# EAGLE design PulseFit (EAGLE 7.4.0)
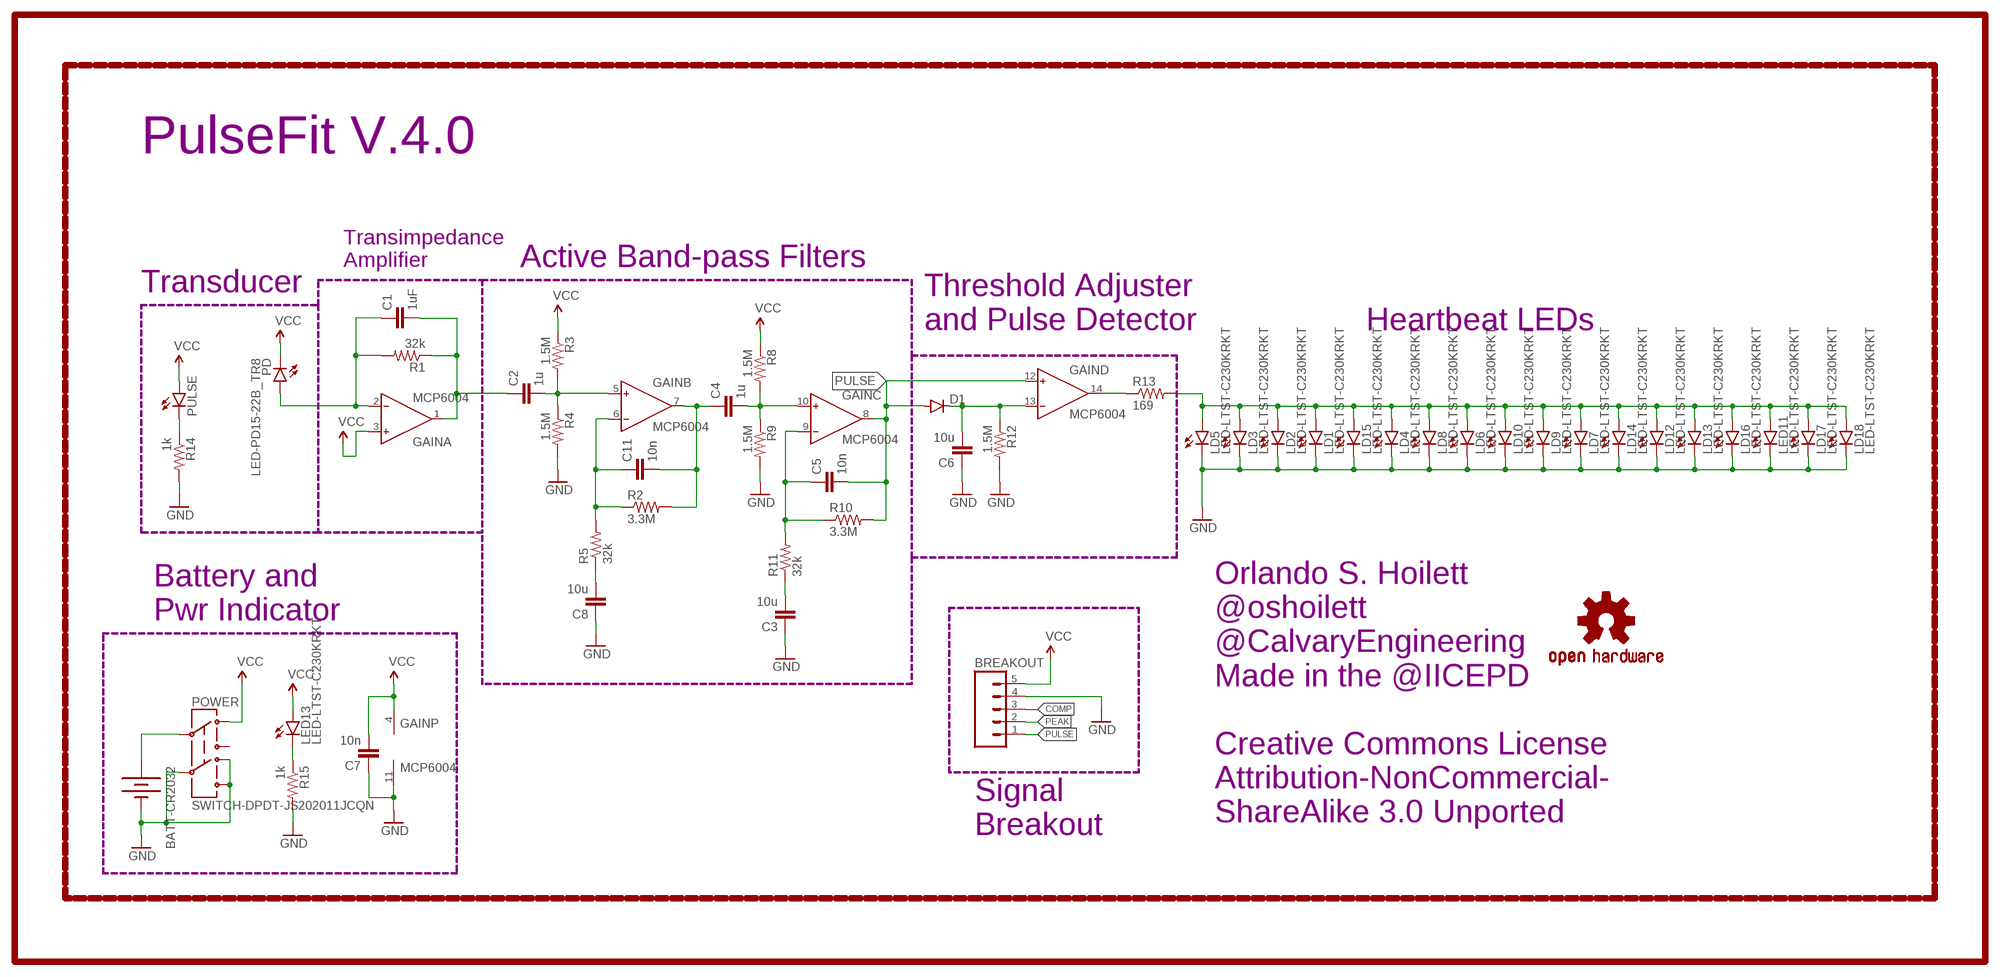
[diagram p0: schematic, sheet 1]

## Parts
BATT-CR2032  BATTERY20SMD  [BATTCON_20MM]
BREAKOUT  M05NO_SILK  [1X05_NO_SILK]
C1  1uF  C-EUC0402  [C0402]
C2  1u  C-EUC0402  [C0402]
C3  10u  C-EUC0805  [C0805]
C4  1u  C-EUC0402  [C0402]
C5  10n  C-EUC0402  [C0402]
C6  10u  C-EUC0805  [C0805]
C7  10n  C-EUC0402  [C0402]
C8  10u  C-EUC0805  [C0805]
C11  10n  C-EUC0402  [C0402]
D1  250mA/100V  DIODEBAS16  [SOD-323]
GAIN  MCP6004  AD8609RU  [TSSOP14]
LD1  LED-LTST-C230KRKT  [LED-1206-BOTTOM]
LD2  LED-LTST-C230KRKT  [LED-1206-BOTTOM]
LD3  LED-LTST-C230KRKT  [LED-1206-BOTTOM]
LD4  LED-LTST-C230KRKT  [LED-1206-BOTTOM]
LD5  LED-LTST-C230KRKT  [LED-1206-BOTTOM]
LD6  LED-LTST-C230KRKT  [LED-1206-BOTTOM]
LD7  LED-LTST-C230KRKT  [LED-1206-BOTTOM]
LD8  LED-LTST-C230KRKT  [LED-1206-BOTTOM]
LD9  LED-LTST-C230KRKT  [LED-1206-BOTTOM]
LD10  LED-LTST-C230KRKT  [LED-1206-BOTTOM]
LD12  LED-LTST-C230KRKT  [LED-1206-BOTTOM]
LD13  LED-LTST-C230KRKT  [LED-1206-BOTTOM]
LD14  LED-LTST-C230KRKT  [LED-1206-BOTTOM]
LD15  LED-LTST-C230KRKT  [LED-1206-BOTTOM]
LD16  LED-LTST-C230KRKT  [LED-1206-BOTTOM]
LD17  LED-LTST-C230KRKT  [LED-1206-BOTTOM]
LD18  LED-LTST-C230KRKT  [LED-1206-BOTTOM]
LED11  LED-LTST-C230KRKT  [LED-1206-BOTTOM]
LED13  LED-LTST-C230KRKT  [LED-1206-BOTTOM]
LOGO1  OSHW-LOGOS  [OSHW-LOGO-S]
PD  LED-PD15-22B_TR8  [LED-PD15-22B_TR8]
POWER  SWITCH-DPDT-JS202011JCQN  [J-LEAD]
PULSE  LED0603  [LED-0603]
R1  32k  R-US_R0402  [R0402]
R2  3.3M  R-US_R0402  [R0402]
R3  1.5M  R-US_R0402  [R0402]
R4  1.5M  R-US_R0402  [R0402]
R5  32k  R-US_R0402  [R0402]
R8  1.5M  R-US_R0402  [R0402]
R9  1.5M  R-US_R0402  [R0402]
R10  3.3M  R-US_R0402  [R0402]
R11  32k  R-US_R0402  [R0402]
R12  1.5M  R-US_R0402  [R0402]
R13  169  R-US_R0402  [R0402]
R14  1k  R-US_R0402  [R0402]
R15  1k  R-US_R0402  [R0402]

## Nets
ANODE: LD1.A LD2.A LD3.A LD4.A LD5.A LD6.A LD7.A LD8.A LD9.A LD10.A LD12.A LD13.A LD14.A LD15.A LD16.A LD17.A LD18.A LED11.A R13.2
COMP: BREAKOUT.3 GAIN.14(D:OUT) R13.1
GND: BATT-CR2032.2(-) BREAKOUT.4 C3.1 C6.1 C7.1 C8.1 GAIN.11(P:V-) LD1.C LD2.C LD3.C LD4.C LD5.C LD6.C LD7.C LD8.C LD9.C LD10.C LD12.C LD13.C LD14.C LD15.C LD16.C LD17.C LD18.C LED11.C POWER.4 POWER.5 POWER.6 R4.2 R9.2 R12.2 R14.2 R15.2
N$1: C1.1 GAIN.2(A:IN-) PD.A-1(A) PD.A-2(A) R1.2
N$2: C1.2 C2.1 GAIN.1(A:OUT) R1.1
N$3: C4.2 GAIN.10(C:IN+) R8.2 R9.1
N$4: C2.2 GAIN.5(B:IN+) R3.2 R4.1
N$5: BATT-CR2032.1(+) POWER.2
N$6: C3.2 R11.1
N$8: C5.1 GAIN.9(C:IN-) R10.1 R11.2
N$9: PULSE.C R14.1
N$10: C11.1 GAIN.6(B:IN-) R2.1 R5.2
N$11: C4.1 C11.2 GAIN.7(B:OUT) R2.2
N$12: LED13.C R15.1
N$14: C8.2 R5.1
PEAK: BREAKOUT.2 C6.2 D1.C GAIN.13(D:IN-) R12.1
PULSE: BREAKOUT.1 C5.2 D1.A GAIN.8(C:OUT) GAIN.12(D:IN+) R10.2
VCC: BREAKOUT.5 C7.2 GAIN.3(A:IN+) GAIN.4(P:V+) LED13.A PD.C-1(C) PD.C-2(C) POWER.1 PULSE.A R3.1 R8.1
Unconnected: POWER.3

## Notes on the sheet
- PulseFit V.4.0
- Transimpedance
  Amplifier
- Active Band-pass Filters
- Transducer
- Threshold Adjuster
  and Pulse Detector
- Heartbeat LEDs
- Battery and
  Pwr Indicator
- Orlando S. Hoilett
  @oshoilett
  @CalvaryEngineering
  Made in the @IICEPD
  
  Creative Commons License
  Attribution-NonCommercial-
  ShareAlike 3.0 Unported
- Signal
  Breakout

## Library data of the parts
BATT-CR2032 = SparkFun-Electromechanical:BATTERY: Battery Holders
BREAKOUT = SparkFun-Connectors:M05: Header 5 Standard 5-pin 0.1" header. Use with straight break away headers (SKU : PRT-00116), right angle break away headers (PRT-00553), swiss pins (PRT-00743), machine pins (PRT-00117), and female headers (PRT-00115). Molex polarized connector foot print use with SKU : PRT-08230 with associated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
C1-C8 C11 = resistor:C-EU: CAPACITOR, European symbol
D1 = SparkFun-DiscreteSemi:DIODE: Diode; PROD_ID: DIO-09646
GAIN = analog-devices:AD8609: Precision Micropower, Low Noise CMOS, Rail-to-Rail Input/Output Operational Amplifiers Source: http://www.analog.com/static/imported-files/data_sheets/AD8603_8607_8609.pdf; MF: ALTERA CORPORATION; MPN: AD8609ARUZ; OC_FARNELL: 1464994; OC_NEWARK: 59K6934
LD1-LD10 LD12-LD18 LED11 LED13 = Orlando:LED-LTST-C230KRKT
LOGO1 = SparkFun-Aesthetics:OSHW-LOGO: Open Source Hardware Logo This logo indicates the piece of hardware it is found on incorporates a OSHW license and/or adheres to the definition of open source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
PD = Orlando:LED-PD15-22B_TR8
POWER = SparkFun-Electromechanical:SWITCH-DPDT-JS202011JCQN
PULSE = SparkFun-LED:LED: LEDs
R1-R5 R8-R15 = resistor:R-US_: RESISTOR, American symbol

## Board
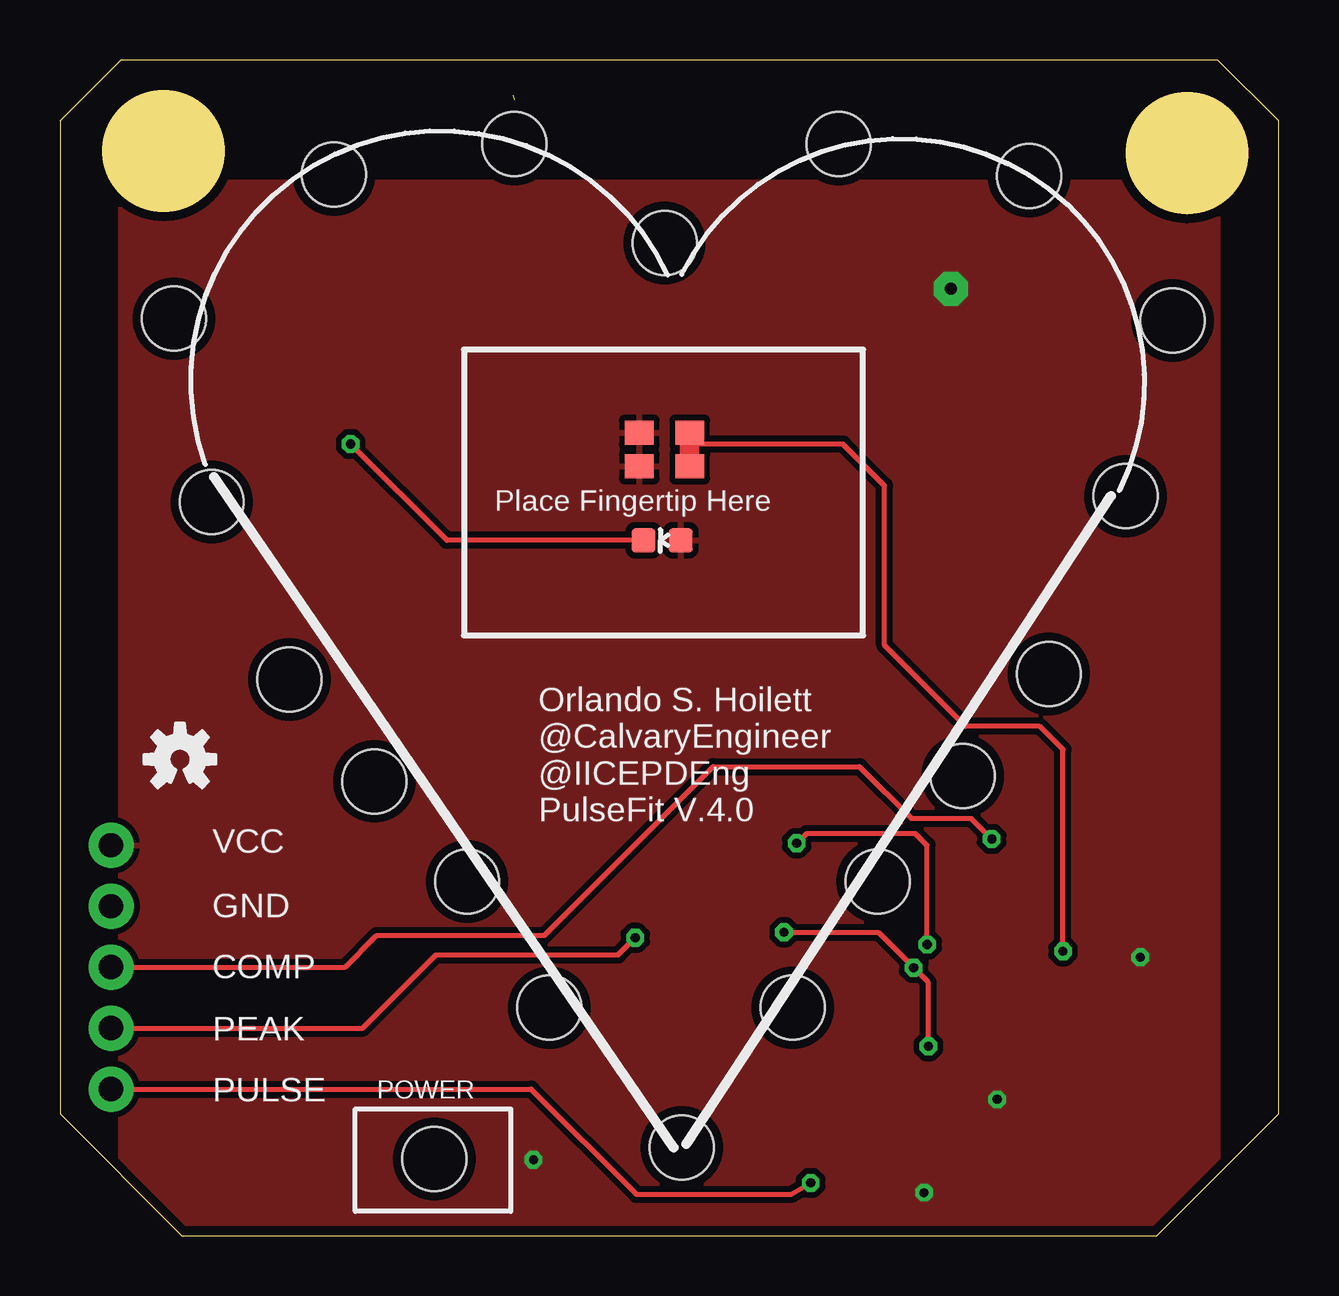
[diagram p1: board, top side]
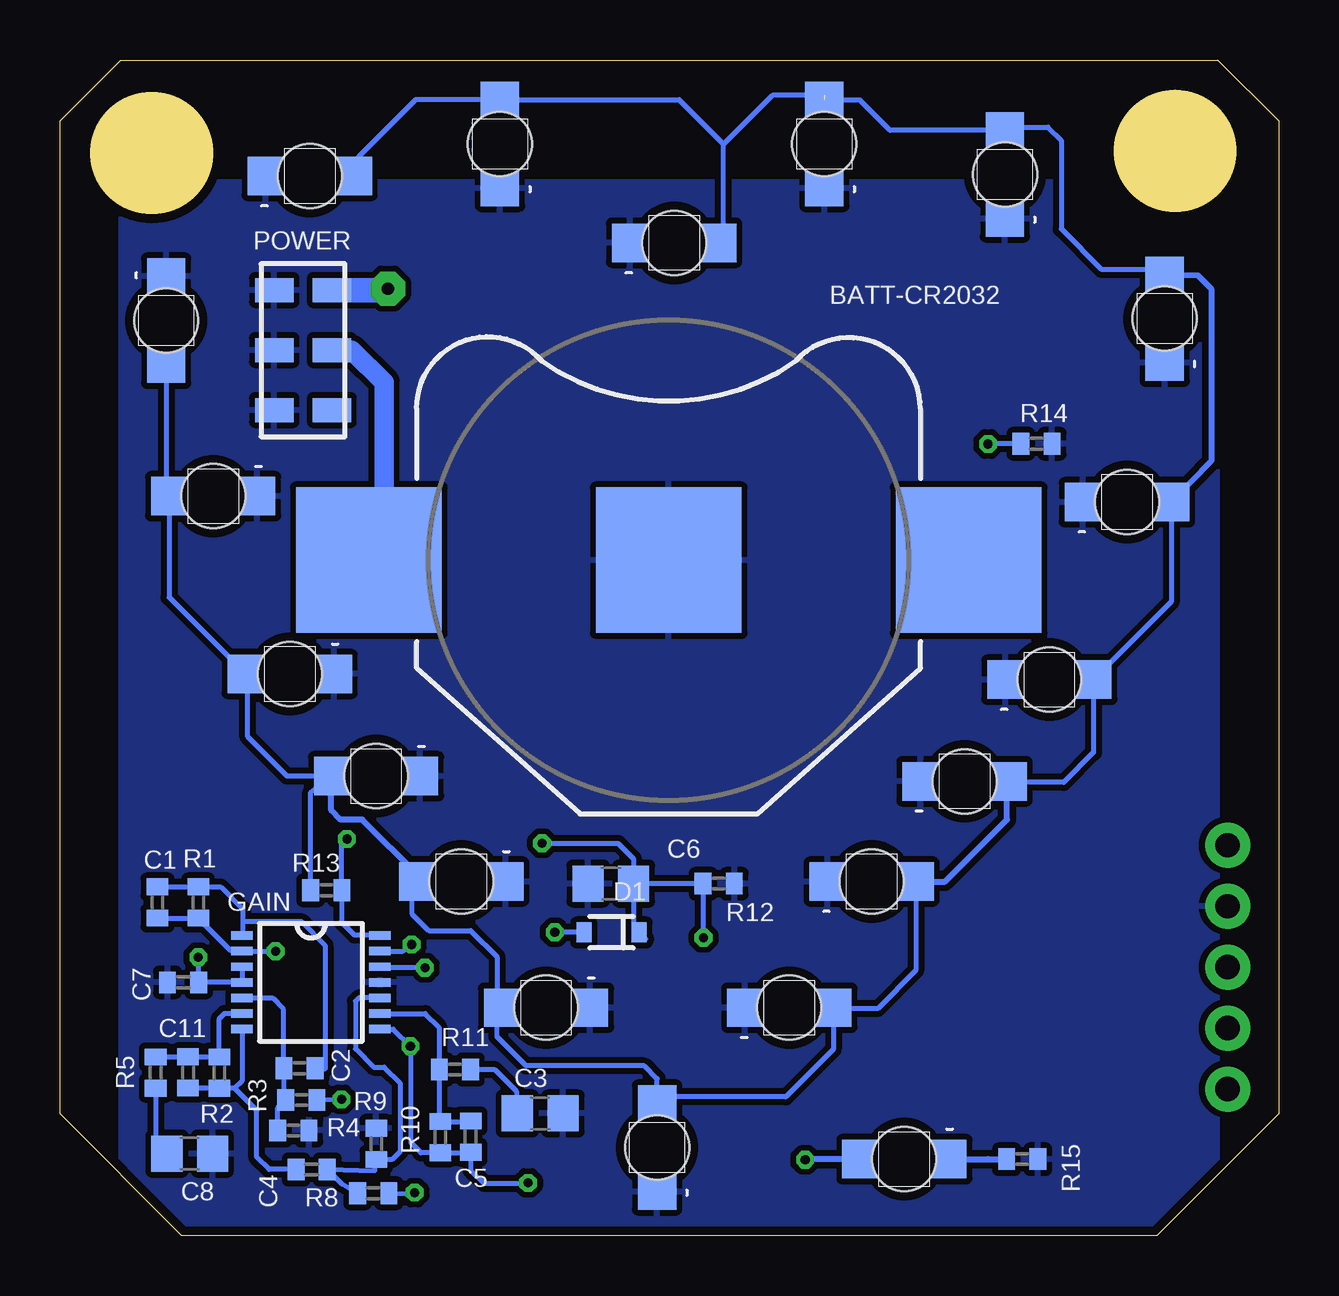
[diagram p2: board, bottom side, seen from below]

Size 50.8 x 49 mm. Coordinates in mm from the lower left corner, seen from the top.
Outline: 4.29,45.21 4.34,45.21
Outline: 46.95,45.12 47,45.12
Outline: 5.08,0 45.72,0 50.8,5.08 50.8,46.46 48.26,49 2.54,49 0,46.46 0,5.08 5.08,0
Copper layers (1*16): Top 0.0356mm / dielectric 1.5011mm / Bottom 0.0356mm
Design rules "LaenPCBOrder": minimum track width 6mil, minimum drill 13mil, track to track 6mil, track to pad 6mil, pad to pad 6mil, via to via 6mil, smd to smd 6mil, copper to edge 15mil, drill to drill 6mil, minimum pad ring 7mil, minimum via ring 7mil, stop-mask expansion 3mil, vias tented up to drill 0mil, thermal gap 10mil

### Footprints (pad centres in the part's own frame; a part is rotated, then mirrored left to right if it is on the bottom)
BATTCON_20MM = smd 6.07 x 6.07: 1 -12.5,0; 2 0,0; 3 12.5,0
1X05_NO_SILK = drill 1.016 pad 1.88: 1 0,0; 2 2.54,0; 3 5.08,0; 4 7.62,0; 5 10.16,0
C0402 = smd 0.7 x 0.9: 1 -0.65,0; 2 0.65,0
C0805 = smd 1.3 x 1.5: 1 -0.95,0; 2 0.95,0
SOD-323 = smd 0.63 x 0.83: A 1.15,0; C -1.15,0
TSSOP14 = smd 0.9 x 0.35: 1 -2.875,1.95; 2 -2.875,1.3; 3 -2.875,0.65; 4 -2.875,0; 5 -2.875,-0.65; 6 -2.875,-1.3; 7 -2.875,-1.95; 8 2.875,-1.95; 9 2.875,-1.3; 10 2.875,-0.65; 11 2.875,0; 12 2.875,0.65; 13 2.875,1.3; 14 2.875,1.95
LED-1206-BOTTOM = smd 1.5 x 1.6: A -1.841,0; C 1.841,0 | hole 2.667: 0,0
LED-PD15-22B_TR8 = smd 1.2 x 1: A-1 -1.05,0.7; A-2 -1.05,-0.7; C-1 1.05,0.7; C-2 1.05,-0.7
J-LEAD = smd 1 x 1.6: 1 -2.5,1.2; 2 0,1.2; 3 2.5,1.2; 4 -2.5,-1.2; 5 0,-1.2; 6 2.5,-1.2
LED-0603 = smd 1 x 1: A 0,-0.677; C 0,0.877
R0402 = smd 0.7 x 0.9: 1 -0.65,0; 2 0.65,0

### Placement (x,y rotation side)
BATT-CR2032  25.43,28.16 0 bottom
BREAKOUT  2.13,6.12 90 top
C1  46.74,13.89 90 bottom
C2  40.82,6.99 180 bottom
C3  30.78,5.11 180 bottom
C4  40.31,2.77 0 bottom
C5  33.68,4.14 270 bottom
C6  27.84,14.68 0 bottom
C7  45.67,10.57 0 bottom
C8  45.39,3.43 180 bottom
C11  45.46,6.81 270 bottom
D1  27.81,12.65 180 bottom
GAIN  40.34,10.57 0 bottom
LD1  25.2,41.38 180 bottom
LD2  32.46,45.5 270 bottom
LD3  40.39,44.16 180 bottom
LD4  46.37,38.14 90 bottom
LD5  44.41,30.82 0 bottom
LD6  41.22,23.41 0 bottom
LD7  37.62,19.16 0 bottom
LD8  34.08,14.77 0 bottom
LD9  30.54,9.51 0 bottom
LD10  25.91,3.68 270 bottom
LD12  16.97,14.77 180 bottom
LD13  13.1,18.94 180 bottom
LD14  9.56,23.18 180 bottom
LD15  6.32,30.58 180 bottom
LD16  4.75,38.22 270 bottom
LD17  11.41,44.23 270 bottom
LD18  18.94,45.5 270 bottom
LED11  20.4,9.51 180 bottom
LED13  15.61,3.2 0 bottom
LOGO1  5,19.86 0 top
PD  25.2,32.77 180 top
POWER  40.67,36.91 270 bottom
PULSE  25.2,28.98 90 top
R1  45.03,13.89 270 bottom
R2  44.16,6.8 270 bottom
R3  40.74,5.66 180 bottom
R4  41.07,4.39 0 bottom
R5  46.81,6.81 90 bottom
R8  37.74,1.78 180 bottom
R9  37.62,3.84 90 bottom
R10  34.95,4.11 270 bottom
R11  34.34,6.93 180 bottom
R12  23.34,14.68 0 bottom
R13  39.7,14.4 180 bottom
R14  10.1,33.01 0 bottom
R15  10.69,3.2 0 bottom

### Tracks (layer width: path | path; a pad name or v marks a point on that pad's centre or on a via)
ANODE  (1 unrouted)
  Bottom 0.203: R13.2 40.35,18.48 LD7.A 41.33,19.16 42.98,20.8 42.98,22.71 43.02,22.75 | 23.11,41.38 LD1.A 23.14,41.39 23.14,45.49 | LD13.A 11,18.9 8.97,18.9 7.72,20.14 LD14.A 4.48,26.42 LD15.A | LED11.A 18.31,9.47 16.71,9.47 15.13,11.06 LD12.A | 18.57,9.48 18.57,7.77 20.55,5.79 25.85,5.79 LD10.A 25.91,6.56 26.44,7.09 31.37,7.09 32.59,8.31 32.59,9.51 LD9.A | 32.26,9.59 LD9.A | LD8.A 36.12,14.61 36.12,13.41 35.43,12.72 33.68,12.72 32.59,11.63 32.59,9.51 LD9.A | LD4.A 46.37,30.91 LD5.A 46.25,26.61 LD6.A | LD16.A 4.76,40.27 7.39,40.27 9.07,41.96 9.07,45.65 9.62,46.2 11.34,46.2 LD17.A 16.2,46.07 17.45,47.32 18.92,47.32 LD18.A | LD3.A 38.35,44.18 38.35,44.96 35.97,47.34 LD2.A 24.99,47.34 23.14,45.49 | 18.91,47.52 21.11,47.52 23.14,45.49
  Bottom 0.254: LD6.A 43.02,22.75 | LD12.A 13.91,14.77 11.33,17.35 11.33,18.91 LD13.A 11.25,18.9 | LD16.A 3.37,40.02 2.82,39.47 2.82,32.28 LD15.A | 23.39,41.38 LD1.A | 18.57,9.48 LED11.A | LD8.A 35.88,15.02 38.2,17.35 39.12,17.35 39.5,17.73 39.5,19.09 LD7.A
COMP  (via drill 0.38)
  Top 0.203: BREAKOUT.3 11.88,11.2 13.21,12.52 20.19,12.52 27.23,19.56 33.33,19.56 35.48,17.4 37.97,17.4 v38.84,16.54
  Bottom 0.203: GAIN.14 37.49,12.55 38.53,12.55 39.05,13.07 R13.1 39.05,16.32 v38.84,16.54
GND
  pour Bottom (isolate 0.254): 48.26,43.92 48.26,0.51 2.54,0.51 2.54,43.92
N$1  (via drill 0.38)
  Top 0.203: v41.81,11.86 41.81,20.27 40.84,21.23 37.74,21.23 34.37,24.61 34.37,31.27 32.64,32.99 26.72,32.99 PD.A-2 | 26.32,33.05 26.25,32.97
  Top 0.813: PD.A-2 26.25,32.97 PD.A-1
  Bottom 0.203: 45.14,13.14 R1.2 | C1.1 R1.2 | v41.81,11.86 v41.81,11.87 GAIN.2 43.66,11.87 R1.2
N$2
  Bottom 0.203: 43.18,13.03 43.18,13.61 44.11,14.54 R1.1 C1.2 | 43.18,13.03 43.18,12.55 GAIN.1 | C2.1 39.75,6.95 39.75,12.12 40.72,13.08 43.13,13.08 43.18,13.03
N$3
  Bottom 0.203: R8.2 39.05,2.16 C4.2 37.68,2.72 R9.1 37.61,3.17 36.96,3.17 36.63,3.5 36.63,6.38 37.29,7.04 37.72,7.04 38.48,7.8 38.48,9.78 38.34,9.92 GAIN.10
N$4
  Bottom 0.203: GAIN.5 41.95,9.92 41.5,9.47 41.5,7.02 C2.2 41.47,5.74 R3.2 41.72,5.33 R4.1
N$5
  Bottom 0.813: POWER.2 38.63,36.91 37.29,35.56 37.29,28.8 BATT-CR2032.1
N$6
  Bottom 0.203: R11.1 32.69,6.93 31.77,6.02 31.77,5.15 C3.2
N$8
  Bottom 0.203: R10.1 33.71,4.76 C5.1 | GAIN.9 35.58,9.27 35,8.69 35,6.95 R11.2 34.99,4.8 R10.1 | 35,4.82 R10.1
N$9  (via drill 0.38)
  Top 0.203: PULSE.C 16.13,28.98 v12.12,32.99
  Bottom 0.203: R14.1 12.1,33.01 v12.12,32.99
N$10
  Bottom 0.203: GAIN.6 43.94,9.27 44.16,9.06 R2.1 C11.1 | C11.1 | C11.1 R5.2
N$11
  Bottom 0.203: GAIN.7 43.21,6.45 43.51,6.15 | 43.51,6.15 44.15,6.15 R2.2 C11.2 | C4.1 42.09,2.77 42.6,3.28 42.6,5.23 43.51,6.15
N$12
  Bottom 0.254: LED13.C 12.11,3.2 R15.1
N$14
  Bottom 0.203: R5.1 46.81,3.9 C8.2
PEAK  (via drill 0.38)
  Top 0.203: v36.14,12.14 36.14,16.28 35.66,16.76 31.12,16.76 v30.71,16.36 | BREAKOUT.2 12.62,8.66 15.67,11.71 23.27,11.71 v23.98,12.42
  Top 0.254: 2.15,8.64 BREAKOUT.2
  Bottom 0.203: C6.2 26.89,12.88 D1.C 26.38,12.37 | GAIN.13 36.5,11.87 v36.14,12.14 | C6.2 R12.1 23.98,14.67 v23.98,12.42 | v30.71,16.36 27.53,16.36 26.9,15.72 26.9,14.69 C6.2
PULSE  (via drill 0.38)
  Top 0.203: v36.2,7.9 36.2,10.57 v35.59,11.18 34.11,12.65 v30.18,12.65 | BREAKOUT.1 19.64,6.12 24.03,1.73 30.48,1.73 v31.29,2.21
  Bottom 0.203: GAIN.8 36.91,8.62 v36.2,7.9 36.17,7.87 36.17,3.89 35.75,3.46 R10.2 33.71,3.46 C5.2 33.68,2.74 33.12,2.18 31.32,2.18 v31.29,2.21 | v35.59,11.18 37.42,11.18 GAIN.12 | D1.A v30.18,12.65
VCC  (via drill 0.38, 0.51 pad 1.42)
  Bottom 0.203: R8.1 36.07,1.75 v36.02,1.8 | GAIN.3 GAIN.4 C7.2 45.02,11.09 v45.03,11.61 | R3.1 v39.07,5.69
  Bottom 0.254: LED13.A 19.74,3.2 v19.74,3.17
  Bottom 1.016: POWER.1 37.2,39.41 v37.13,39.47
  pour Top (isolate 0.254): 2.54,43.92 48.26,43.92 48.26,0.51 2.54,0.51

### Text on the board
tNames: Orlando S. Hoilett / @CalvaryEngineer / @IICEPDEng / PulseFit V.4.0 | VCC | GND | COMP | PEAK | PULSE | POWER
tplace-old: Creative Commons License / Attribution-NonCommercial- / ShareAlike 3.0 Unported
_tsilk: Place Fingertip Here

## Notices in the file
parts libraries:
SparkFun-Aesthetics: Licensing: Creative Commons ShareAlike 4.0 International - https://creativecommons.org/licenses/by-sa/4.0
